FUNCTION_BLOCK FB_Configure
VAR_INPUT
	


	nStartModeSelect	:	INT := 1;
	nCamId				:	UDINT := 1;
	refMasterAxis		:	REFERENCE TO AXIS_REF;
	
	MinSoftLimit		:	LREAL;
	MaxSoftLimit		:	LREAL;
	MaxVelocity			:	LREAL;
END_VAR
VAR_OUTPUT
END_VAR
VAR
END_VAR

END_FUNCTION_BLOCK
